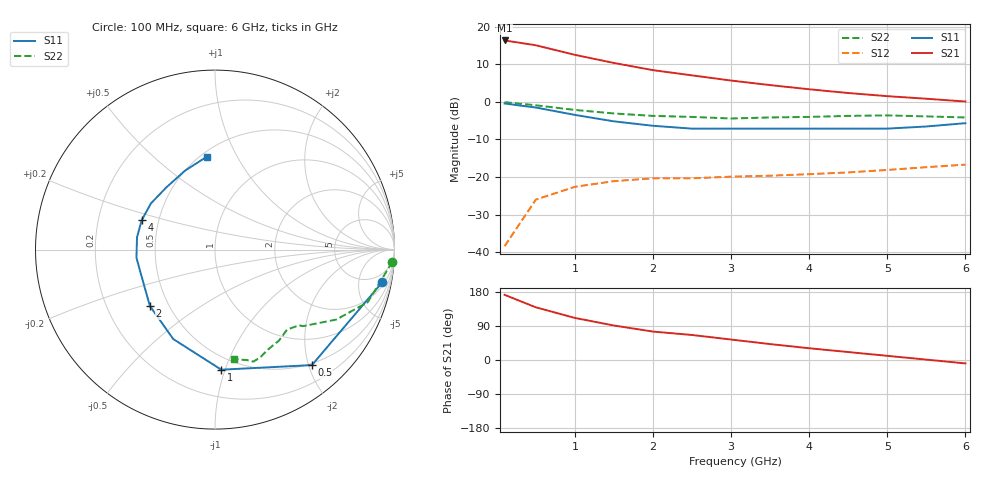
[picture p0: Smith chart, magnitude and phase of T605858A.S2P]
!AT-60585
!S AND NOISE PARAMETERS at Vce=8V  Ic=2mA.  LAST UPDATED 07-21-92
# ghz s ma r 50
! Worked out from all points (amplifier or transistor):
!   13 points, 100 MHz to 6 GHz, reference 50 ohm
!   highest |S21| = 16.3 dB at 100 MHz (marker M1)
!   |S21| within 3 dB of that: start of sweep to 836.9 MHz
!   unconditionally stable (mu >= 1): 2.218 GHz to end of sweep
!   at 1 GHz: K = 0.49, MSG = 17.6 dB, |S12| = -22.6 dB
!   at 3 GHz: K = 1.27, MAG = 9.7 dB, |S12| = -19.9 dB
!   at 6 GHz: K = 1.28, MAG = 5.2 dB, |S12| = -16.7 dB
!   lowest NFmin = 1.40 dB at 1 GHz
!   S11 on the Smith chart (normalised r, x): 100 MHz: 3, -10; 500 MHz: 0.47, -2.06; 1 GHz: 0.40, -0.97; 2 GHz: 0.39, -0.32; 4 GHz: 0.40, +0.16; 6 GHz: 0.54, +0.76
0.1  0.95 -11.0  6.56 172.0  0.012 82.0  0.99 -4.0
0.5  0.84 -50.0  5.66 139.0  0.05 61.0  0.9 -19.0
1  0.67 -87.0  4.22 111.0  0.074 43.0  0.78 -30.0
1.5  0.55 -115.0  3.29 91.0  0.088 36.0  0.7 -36.0
2  0.48 -139.0  2.64 75.0  0.096 30.0  0.65 -41.0
2.5  0.44 -155.0  2.25 66.0  0.096 32.0  0.63 -42.0
3  0.44 -174.0  1.92 54.0  0.101 32.0  0.6 -48.0
3.5  0.44 171.0  1.67 42.0  0.104 28.0  0.62 -55.0
4  0.44 158.0  1.47 31.0  0.109 30.0  0.63 -62.0
4.5  0.44 144.0  1.31 21.0  0.115 30.0  0.65 -67.0
5  0.44 128.0  1.19 11.0  0.124 30.0  0.66 -71.0
5.5  0.47 111.0  1.1 1.0  0.135 30.0  0.64 -74.0
6  0.52 95.0  1.01 -9.0  0.146 28.0  0.62 -80.0
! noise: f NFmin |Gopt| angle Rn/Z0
1  1.4  0.5  53  0.32
2  1.9  0.42  108  0.34
4  2.9  0.4  -144  0.46
